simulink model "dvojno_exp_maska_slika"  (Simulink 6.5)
settings: Solver=FixedStepDiscrete  StartTime=0.0  StopTime=50e-6  RelTol=1e-6
undefined symbols (not defined in the file or in its folder): blocks, Discrete, powergui, ZData
libraries: powerlib x6

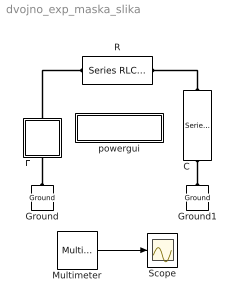
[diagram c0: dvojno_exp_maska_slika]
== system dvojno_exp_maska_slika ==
  C : powerlib/Elements/Series RLC Branch  Orientation=down  DialogController=PMDialogs.PMDefaultMaskDlg  PhysicalDomain=powersysdomain  SubClassName=unknown  LeftPortType=p1  RightPortType=p1  LConnTagsString=__new0  RConnTagsString=__new0  BranchType=C  Resistance=1  Inductance=1e-3  SetiL0=off  InitialCurrent=0  Capacitance=10e-9  Setx0=on  InitialVoltage=0  Measurements=Branch voltage
  E : Subsystem  Orientation=up  mask(Impulsen generator){UM=100e3, Tc=1.2e-6, Tz=50e-6}
      mask prompts: UM "Maksimalen napon (V)"; Tc "Vreme na celoto (s)"; Tz "Vreme na grbot (s)"
      mask help: So ovoj element e definiran idealen naponski generator so dvoen eksponencijalen oblik.
      mask init:
      | a = 0.69 / Tz;
      | b = 3.24 / Tc;
      | k = (a/b)^(-a/(a-b)) -  (a/b)^(-b/(a-b));
      | Um = UM / k;
  Ground : powerlib/Elements/Ground  Orientation=down  DialogController=PMDialogs.PMDefaultMaskDlg  PhysicalDomain=powersysdomain  SubClassName=unknown  LeftPortType=p1  RightPortType=p1  LConnTagsString=a
  Ground1 : powerlib/Elements/Ground  Orientation=down  DialogController=PMDialogs.PMDefaultMaskDlg  PhysicalDomain=powersysdomain  SubClassName=unknown  LeftPortType=p1  RightPortType=p1  LConnTagsString=a
  Multimeter : powerlib/Measurements/Multimeter  SystemSampleTime=-1  PhasorSimulation=off  OutputType=Complex  sel=[2 1]  L=2  Gain=[1 1]  yselected={'Usrc: E/Kontrolirano E','Ub: C'};  PSBOutputType=1  PSBequivalent=0  AxesSetting=[0,0.1,-100,100]  Display=0  SavedBlockNames=-11
  R : powerlib/Elements/Series RLC Branch  DialogController=PMDialogs.PMDefaultMaskDlg  PhysicalDomain=powersysdomain  SubClassName=unknown  LeftPortType=p1  RightPortType=p1  LConnTagsString=__new0  RConnTagsString=__new0  BranchType=R  Resistance=100  Inductance=1e-3  SetiL0=on  InitialCurrent=0  Capacitance=1e-6  Setx0=off  InitialVoltage=0  Measurements=None
  Scope : Scope
  powergui : Subsystem  AncestorBlock=powerlib/powergui  InitFcn=powergui( 'InitFcn_Callback' , gcb , 0 , [ ] );  mask(PSB option menu block){SimulationMode=Discrete, SampleTime=0.05e-6, echomessages=off, RestoreLinks=warning, x0status=blocks, Frange=[0:2:500], Ylog=off, Xlog=on, ShowGrid=off, save=off, variable=ZData, structure=, ZoomFFT=on, StartTime=0.0, cycles=1, DisplayStyle=1, fundamental=60, FreqAxis=off, MaxFrequency=1000, frequencyindice=0, frequencyindicesteady=1, RmsSteady=1, display=off, Ts=0, frequency=60, methode=off, HookPort=off, Interpol=off}
      mask prompts: SimulationMode "Simulation mode"; SampleTime "Sample time Ts (when simulation mode is Discrete) (s)"; echomessages "Echo  Messages"; RestoreLinks "Restore disabled links"; x0status "Initial electrical states status"; Frange "Impedance tool: Frequency Range"; Ylog "Impedance tool: Log impedance"; Xlog "Impedance tool: log Frequency"; ShowGrid "Impedance tool: grid"; save "Impedance tool: Save Data To Workspace"; variable "Impedance tool: Variable Name"; structure "Structure Name (PSBFFTSCOPE)"; ZoomFFT "ZoomFFT (PSBFFTSCOPE)"; StartTime "Start Time (PSBFFTSCOPE)"; cycles "Cycles (PSBFFTSCOPE)"; DisplayStyle "Display style (PSBFFTSCOPE)"; fundamental "Fundamental (PSBFFTSCOPE)"; FreqAxis "Frequency Axis (PSBFFTSCOPE)"; MaxFrequency "Max Frequency (PSBFFTSCOPE)"; frequencyindice "Load flow frequency (Hz)"; frequencyindicesteady "Frequency indice (STEADYSTATE)"; RmsSteady "RMS display (STEADYSTATE)"; display "Display Results"; Ts "OBSOLETE 1"; frequency "Phasor frequency (Hz)"; methode "Phasor simulation"; HookPort "Hook port"; Interpol "Interpolate"
      mask init:
      | powerlibroot = which('powersysdomain');
      | PSBroot = powerlibroot(1:end-16);
      | %
      | switch SimulationMode
      | 	case 1
      | 		message=sprintf('Continuous');
      | 	case 2
      |         SampleTimeeval=evalin('base',SampleTime,'NaN');
      |         if isnan(SampleTimeeval)
      |             message=sprintf('Warning !!,\nUndefined sample time');
      |         else
      |             message=sprintf('Discrete,\nTs = %.4g s.',SampleTimeeval);
      |         end
      | 	case 3
      | 		message=sprintf('Phasors');
      | end
      | if strcmp(bdroot,'powerlib')
      |   message='powergui';
      | end
      | power_initmask();
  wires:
  Multimeter/1 -> Scope/1
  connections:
  C/LConn1 -- R/RConn1
  Ground1/LConn1 -- C/RConn1
  Ground/LConn1 -- E/LConn1
  E/RConn1 -- R/LConn1

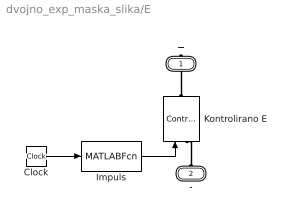
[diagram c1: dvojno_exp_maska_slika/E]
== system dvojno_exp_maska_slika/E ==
  Clock : Clock
  Impuls : MATLABFcn  MATLABFcn=Um*(exp(-a*u)-exp(-b*u))  OutputSignalType=real
  Kontrolirano E : powerlib/Electrical Sources/Controlled Voltage Source  Orientation=up  DialogController=PMDialogs.PMDefaultMaskDlg  SystemSampleTime=-1  Initialize=on  Source_Type=AC  Amplitude=0  Phase=0  Frequency=0  Measurements=Voltage
  + : PMIOPort  Orientation=down  Port=1  Side=Right
  - : PMIOPort  Orientation=up  Port=2  Side=Left
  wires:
  Impuls/1 -> Kontrolirano E/1
  Clock/1 -> Impuls/1
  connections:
  +/RConn1 -- Kontrolirano E/RConn1
  -/RConn1 -- Kontrolirano E/LConn1

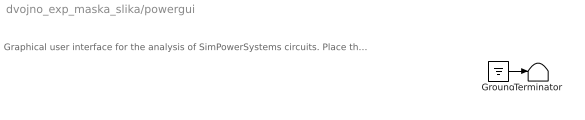
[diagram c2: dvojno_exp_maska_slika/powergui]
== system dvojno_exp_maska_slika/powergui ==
  note: Graphical user interface for the analysis of SimPowerSystems circuits. Place the Powergui block in the top-level of your model and double-click on it to open the GUI.
  Ground : Ground
  Terminator : Terminator
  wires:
  Ground/1 -> Terminator/1
